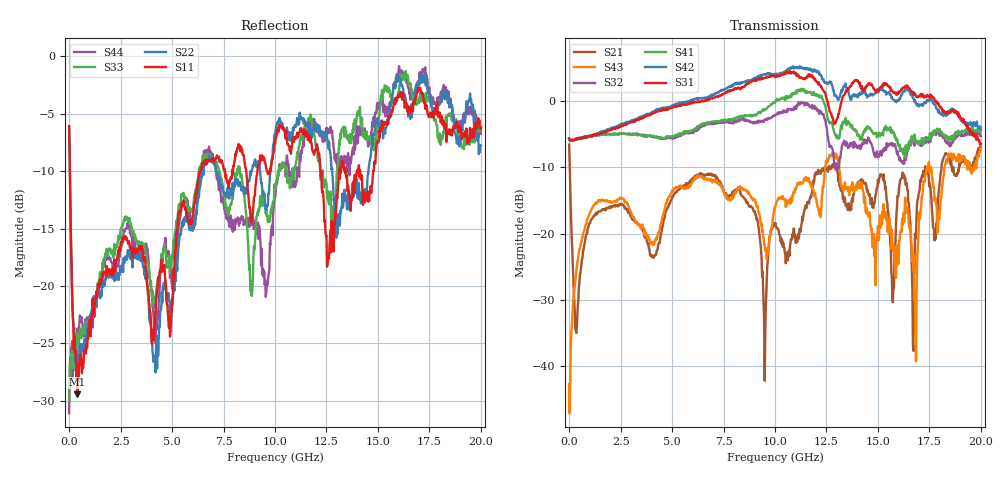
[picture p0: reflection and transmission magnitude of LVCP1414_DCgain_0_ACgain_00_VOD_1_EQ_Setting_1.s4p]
!Agilent Technologies,N5230A,MY46400459,A.07.50.48
!Agilent N5230A: A.07.50.48
!Date: Tuesday, April 17, 2012 18:26:01
!Correction: S11(Full 4 Port(1,2,3,4))
!S12(Full 4 Port(1,2,3,4))
!S13(Full 4 Port(1,2,3,4))
!S14(Full 4 Port(1,2,3,4))
!S21(Full 4 Port(1,2,3,4))
!S22(Full 4 Port(1,2,3,4))
!S23(Full 4 Port(1,2,3,4))
!S24(Full 4 Port(1,2,3,4))
!S31(Full 4 Port(1,2,3,4))
!S32(Full 4 Port(1,2,3,4))
!S33(Full 4 Port(1,2,3,4))
!S34(Full 4 Port(1,2,3,4))
!S41(Full 4 Port(1,2,3,4))
!S42(Full 4 Port(1,2,3,4))
!S43(Full 4 Port(1,2,3,4))
!S44(Full 4 Port(1,2,3,4))
!S4P File: Measurements: <S11,S12,S13,S14>,
!<S21,S22,S23,S24>,
!<S31,S32,S33,S34>,
!<S41,S42,S43,S44>:
# Hz S  dB  R 50
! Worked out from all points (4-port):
!   801 points, 300 kHz to 20 GHz, reference 50 ohm
!   strongest paths, dB at 300 kHz, 5 GHz, 10 GHz, 15 GHz, 20 GHz:
!     S31: -5.6, -0.9, 3.7, 1.6, -6.4
!     S42: -5.7, -0.6, 4.1, 1.8, -4.2
!     S41: -5.7, -5.3, -0.2, -4.9, -4.4
!     S32: -5.6, -5.6, -2.1, -8.5, -5.3
!     S43: -42.8, -13.5, -16.2, -18.9, -7.1
!     S21: -6.5, -14.5, -18.9, -11.8, -7.0
!   lowest |S11| = -29.4 dB at 400.3 MHz (marker M1), VSWR 1.07, Z = 53.1 + j1.58 ohm
!   |S11| at or under -10 dB: 37.58 MHz to 6.369 GHz (6.332 GHz wide, 198 % of centre); 12.21 GHz to 13.12 GHz (906.3 MHz wide, 7.16 % of centre); 14.13 GHz to 14.77 GHz (640.9 MHz wide, 4.43 % of centre)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
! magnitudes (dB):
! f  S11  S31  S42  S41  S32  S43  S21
! 300 kHz  -6.1  -5.6  -5.7  -5.7  -5.6  -42.8  -6.5
! 400.3 MHz  -29.4  -5.6  -5.6  -5.7  -5.7  -24.2  -32.4
! 9.975 GHz  -7.6  3.8  4.1  -0.1  -2.2  -16.1  -18.5
! 12.88 GHz  -14.5  -3.4  1.2  -4.7  -9.3  -8.0  -9.7
! 16.8 GHz  -3.7  1.0  0.2  -5.6  -5.9  -30.3  -20.1
! 17.4 GHz  -4.9  1.0  0.3  -5.7  -5.6  -9.8  -10.5
! 20 GHz  -6.2  -6.4  -4.2  -4.4  -5.3  -7.1  -7.0
